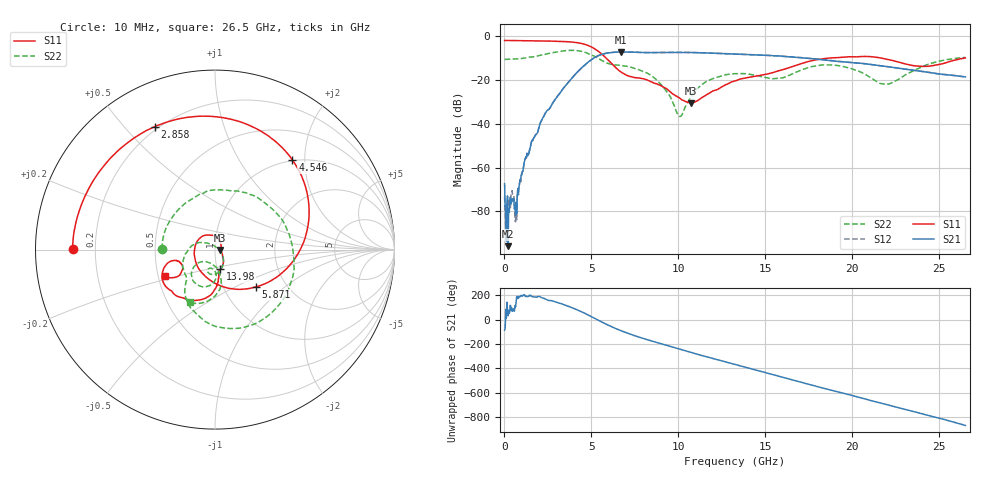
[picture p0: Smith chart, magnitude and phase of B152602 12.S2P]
!  2-Port S-parameters saved by WinCal
! VAR MeasName=S-Parameters (CALIBRATED_DATA) read from VNA (N5242A)
! VAR MeasDate=2016-1-5 16:27:07
! VAR NAME=B152602 12
! VAR FILENAME=B152602 12.S2P
! VAR DATE=2016-1-5 16:27:07
! VAR PHYS_PORTS=1,2
# Hz S DB R 50
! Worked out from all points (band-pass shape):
!   801 points, 10 MHz to 26.5 GHz, reference 50 ohm
!   highest |S21| = -7.26 dB at 6.699 GHz (marker M1); lowest = -95.9 dB at 208.7 MHz (marker M2)
!   |S21| within 3 dB of the highest: 5.089 GHz to 17.61 GHz (12.52 GHz wide, 110 % of centre)
!   lowest |S11| = -30.6 dB at 10.74 GHz (marker M3), VSWR 1.06, Z = 53 - j0.232 ohm
!   |S11| at or under -10 dB: 5.839 GHz to 18.73 GHz (12.9 GHz wide, 105 % of centre); 21.62 GHz to 26.5 GHz (4.878 GHz wide, 20.3 % of centre)
!   |S22| runs from -36.7 to -6.5 dB; largest |S21 - S12| = 0.0029
!   S11 on the Smith chart (normalised r, x): 10 MHz: 0.12, +0.00; 2.858 GHz: 0.19, +0.61; 4.546 GHz: 0.99, +1.74; 5.871 GHz: 1.41, -0.65; 13.98 GHz: 1.04, -0.23; 26.5 GHz: 0.54, -0.18
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1e7  -2.01 179.7  -67.39 -86.2  -73.40 -14.3  -10.67 179.4
2.08675e8  -2.02 175.7  -95.90 32.8  -81.79 87.2  -10.58 167.3
7.053625e8  -2.07 165.5  -80.93 -168.8  -83.78 177.0  -10.44 137.2
1.102712e9  -2.13 157.3  -59.39 -158.0  -59.47 -161.5  -10.15 114.1
1.566288e9  -2.18 147.6  -47.94 -165.9  -47.88 -166.5  -9.53 85.7
2.857675e9  -2.35 116.1  -29.56 149.7  -29.58 149.8  -7.48 10.6
4.447075e9  -3.41 54.6  -14.44 64.3  -14.45 64.4  -7.03 -80.5
4.546412e9  -3.61 49.1  -13.72 58.0  -13.73 58.0  -7.23 -85.7
5.142438e9  -5.60 11.9  -10.00 15.5  -10.00 15.6  -9.10 -113.1
5.870912e9  -10.25 -42.6  -7.82 -38.1  -7.80 -38.1  -12.24 -131.5
6.698725e9  -16.41 -116.4  -7.26 -90.1  -7.27 -90.1  -13.46 -143.1
8.851038e9  -22.17 95.9  -7.52 168.6  -7.51 168.5  -20.82 154.1
1.004309e10  -28.09 28.2  -7.48 118.9  -7.46 119.0  -36.57 67.8
1.073845e10  -30.55 -4.2  -7.51 90.4  -7.50 90.4  -27.49 -32.0
1.3255e10  -20.47 -62.9  -8.19 -8.2  -8.19 -8.2  -17.16 -93.5
1.398348e10  -18.93 -74.5  -8.42 -36.3  -8.42 -36.3  -17.28 -104.2
1.56391e10  -16.16 -82.0  -9.00 -99.6  -9.00 -99.7  -19.38 -99.4
1.769208e10  -11.21 -100.9  -10.33 -178.6  -10.29 -178.5  -13.92 -97.7
1.977816e10  -9.46 -131.3  -11.99 104.7  -11.97 104.2  -14.48 -134.2
2.209604e10  -10.75 -162.1  -14.09 17.5  -14.05 17.1  -21.83 -103.2
2.421524e10  -13.90 -154.0  -16.38 -61.0  -16.37 -61.2  -13.31 -82.2
2.65e10  -10.00 -151.8  -18.64 -149.2  -18.63 -149.4  -9.76 -115.6
